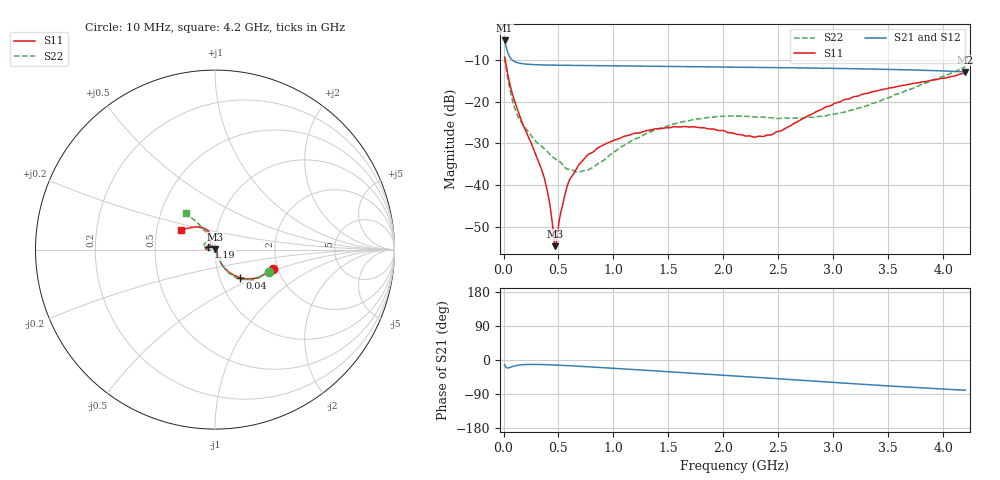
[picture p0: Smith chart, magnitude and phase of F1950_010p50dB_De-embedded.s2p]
! Integrated Device Technology
! Corporate Headquarters
! 6024 Silver Creek Valley Road
! San Jose, CA 95138  USA
! Phone:  1-408-284-8200
! Toll Free:  1-800-223-1366
! Webpage:  http://www.idt.com/
! Timing and RF Division
! 515 Groton Road, Suite 102
! Westford, MA 01886-6024
! Device:  F1950
! Description: 7-bit 0.25 dB Digital Step Attenuator
! Frequency:  150.0 -  4000.00 MHz
! Package:  4x4 mm Thin QFN Plastic Package: 24 pin
! Ports:  2 RF, 12 DC
!  Pin  1  = D0
!  Pin  2  = VDD
!  Pin  3  = Vmode
!  Pin  4  = GND
!  Pin  5  = RF1  =  Port 1
!  Pin  6  = GND
!  Pin  7  = GND
!  Pin  8  = GND
!  Pin  9  = GND
!  Pin 10  = GND
!  Pin 11  = GND
!  Pin 12  = GND
!  Pin 13  = GND
!  Pin 14  = RF2  =  Port 2
!  Pin 15  = GND
!  Pin 16  = LE
!  Pin 17  = CLK
!  Pin 18  = DATE
!  Pin 19  = D6
!  Pin 20  = D5
!  Pin 21  = D4
!  Pin 22  = D3
!  Pin 23  = D2
!  Pin 24  = D1
! State:  42
! Atten State:  10.50 dB
! Voltage:  +5.00 Volts
! Current:  Not Measured mA
! Data:  The device was measured on a the F195X evaluation board which has
!  individual transmission lines to the RF pins.  Data was collected
!  using a calibrated network analyzer.  The evaluation board was
!  de-embedded using a TRL calibration technique.
!  The reference plane is the edge of the package pin.
! Misc:  Board 2019
!  Action Tracker AT0250
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# GHz S dB R 50
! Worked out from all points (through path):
!   420 points, 10 MHz to 4.2 GHz, reference 50 ohm
!   highest |S21| = -5.44 dB at 10 MHz (marker M1); lowest = -12.9 dB at 4.2 GHz (marker M2)
!   group delay of S21, straight-line fit = 48.8 ps
!   lowest |S11| = -54.5 dB at 470 MHz (marker M3), VSWR 1.00, Z = 50.2 + j0.0885 ohm
!   |S11| at or under -10 dB: 14.47 MHz to end of sweep
!   |S22| runs from -36.9 to -9.7 dB; largest |S21 - S12| = 0.00036
!   S11 on the Smith chart (normalised r, x): 10 MHz: 1.87, -0.46; 40 MHz: 1.24, -0.40; 1.19 GHz: 0.92, +0.03; 4.2 GHz: 0.67, +0.15
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0.01  -9.41 -18.6  -5.44 -12.5  -5.44 -12.5  -9.66 -22.8
0.04  -13.66 -48.6  -8.43 -21.1  -8.43 -21.1  -14.70 -54.9
0.09  -19.02 -63.3  -10.31 -16.5  -10.31 -16.5  -20.59 -64.1
0.14  -22.91 -66.0  -10.83 -13.5  -10.83 -13.5  -24.00 -66.4
0.36  -37.30 -52.7  -11.28 -12.1  -11.28 -12.1  -30.97 -74.0
0.41  -42.84 -46.4  -11.31 -12.5  -11.30 -12.6  -32.24 -75.1
0.45  -50.43 -22.1  -11.33 -13.0  -11.33 -13.0  -33.30 -80.2
0.47  -54.47 27.8  -11.33 -13.3  -11.33 -13.3  -33.66 -83.6
0.49  -51.61 83.2  -11.34 -13.5  -11.34 -13.5  -33.95 -85.9
0.53  -45.42 113.7  -11.36 -14.1  -11.36 -14.1  -34.82 -88.6
0.59  -39.32 123.8  -11.38 -15.0  -11.38 -15.0  -36.15 -101.6
0.71  -34.36 133.2  -11.42 -16.9  -11.41 -16.9  -36.64 -126.3
0.88  -30.74 143.3  -11.47 -19.8  -11.46 -19.8  -34.50 -158.6
1.19  -27.58 158.6  -11.56 -25.2  -11.55 -25.3  -28.98 176.5
1.41  -26.48 168.3  -11.61 -29.3  -11.61 -29.3  -26.46 168.6
1.73  -26.00 175.8  -11.70 -35.1  -11.70 -35.1  -24.28 160.3
2.11  -27.72 168.1  -11.80 -42.3  -11.80 -42.3  -23.50 150.5
2.43  -27.98 134.1  -11.90 -48.2  -11.90 -48.2  -23.85 140.1
2.81  -22.92 108.7  -12.02 -55.5  -12.02 -55.5  -23.77 124.3
3.1  -19.54 110.2  -12.14 -61.0  -12.14 -61.1  -22.52 118.1
3.51  -16.77 121.3  -12.35 -68.6  -12.34 -68.6  -19.04 117.7
4.2  -13.15 150.2  -12.93 -79.6  -12.92 -79.7  -11.74 128.3
